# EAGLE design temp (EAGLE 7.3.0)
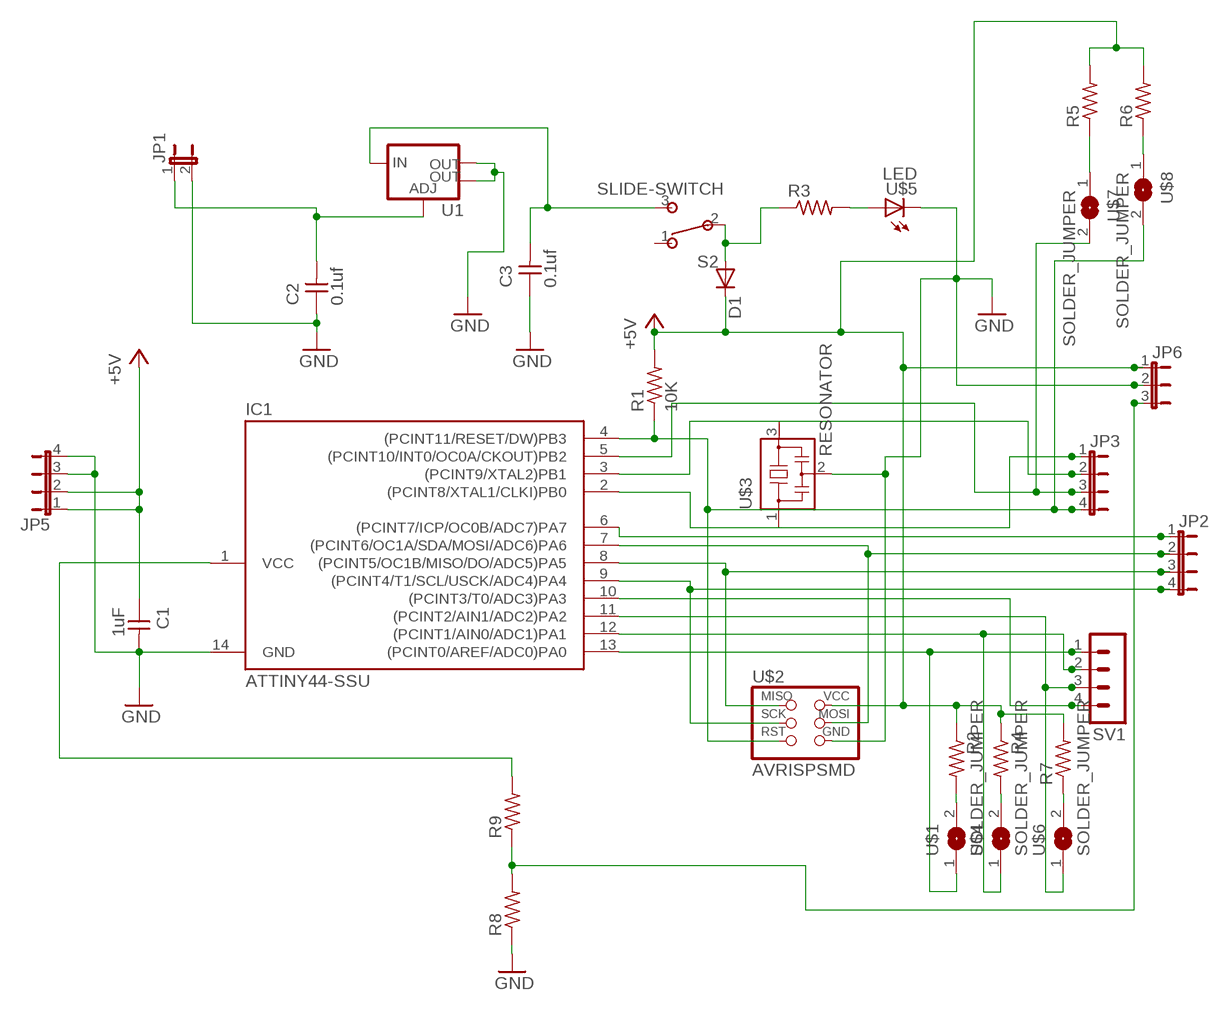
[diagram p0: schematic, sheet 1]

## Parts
C1  1uF  CAP-UNPOLARIZED  [C1206]
C2  0.1uf  CAP-UNPOLARIZED  [C1206]
C3  0.1uf  CAP-UNPOLARIZED  [C1206]
D1  DIODESOD123  [SOD123]
IC1  ATTINY44-SSU  [SOIC14]
JP1  JP1E  [JP1]
JP2  JP4E  [JP4]
JP3  JP4E  [JP4]
JP5  JP4E  [JP4]
JP6  JP2W  [JP2W]
R1  10K  RES-US1206  [R1206]
R2  RES-US1206FAB  [R1206FAB]
R3  RES-US1206  [R1206]
R4  RES-US1206FAB  [R1206FAB]
R5  RES-US1206FAB  [R1206FAB]
R6  RES-US1206FAB  [R1206FAB]
R7  RES-US1206FAB  [R1206FAB]
R8  RES-US1206FAB  [R1206FAB]
R9  RES-US1206FAB  [R1206FAB]
S2  SLIDE-SWITCH  [AYZ0102AGRLC]
SV1  MA04-1  [MA04-1]
U1  V_REG_LM1117SOT223  [SOT223]
U$1  SOLDER_JUMPER  [SJFAB]
U$2  AVRISPSMD  [2X03SMD]
U$3  RESONATOR  [EFOBM]
U$4  SOLDER_JUMPER  [SJFAB]
U$5  LED  [LED1206]
U$6  SOLDER_JUMPER  [SJFAB]
U$7  SOLDER_JUMPER  [SJFAB]
U$8  SOLDER_JUMPER  [SJFAB]

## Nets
+5V: C1.1 D1.CATHODE(C) IC1.1(VCC) JP5.1 JP5.2 JP6.1 R1.2 R2.1 R4.1 R5.2 R6.2 R7.2 R9.2 U$2.2(VCC)
GND: C1.2 C2.1 C3.1 IC1.14(GND) JP1.2 JP5.3 JP5.4 JP6.2 R8.1 U1.2(OUT) U1.4(OUT) U$2.6(GND) U$3.2 U$5.2(C)
N$1: IC1.2((PCINT8/XTAL1/CLKI)PB0) JP3.1 U$3.1
N$2: IC1.8((PCINT5/OC1B/MISO/DO/ADC5)PA5) JP2.3 U$2.1(MISO)
N$3: IC1.3((PCINT9/XTAL2)PB1) JP3.2 U$3.3
N$4: IC1.5((PCINT10/INT0/OC0A/CKOUT)PB2) JP3.3 U$7.2
N$5: IC1.4((PCINT11/RESET/DW)PB3) JP3.4 R1.1 U$2.5(RST) U$8.2
N$6: IC1.9((PCINT4/T1/SCL/USCK/ADC4)PA4) JP2.4 U$2.3(SCK)
N$7: IC1.7((PCINT6/OC1A/SDA/MOSI/ADC6)PA6) JP2.2 U$2.4(MOSI)
N$8: IC1.13((PCINT0/AREF/ADC0)PA0) SV1.1 U$1.1
N$9: IC1.12((PCINT1/AIN0/ADC1)PA1) SV1.2 U$4.1
N$10: IC1.11((PCINT2/AIN1/ADC2)PA2) SV1.3 U$6.1
N$11: IC1.10((PCINT3/T0/ADC3)PA3) SV1.4
N$12: C2.2 JP1.1 U1.1(ADJ)
N$13: C3.2 S2.3 U1.3(IN)
N$14: IC1.6((PCINT7/ICP/OC0B/ADC7)PA7) JP2.1
N$15: JP6.3 R8.2 R9.1
N$16: D1.ANODE(A) R3.1 S2.2
N$17: R3.2 U$5.1(A)
N$18: R2.2 U$1.2
N$19: R5.1 U$7.1
N$20: R6.1 U$8.1
N$21: R4.2 U$4.2
N$22: R7.1 U$6.2
Unconnected: S2.1

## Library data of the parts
C1-C3 = fab:CAP-UNPOLARIZED
D1 = fab:DIODE: DIODE
IC1 = fab:ATTINY44
JP1 = jumper:JP1E: JUMPER
JP2 JP3 JP5 = jumper:JP4E: JUMPER
JP6 = jumper:JP2W: JUMPER
R1-R9 = fab:RES-US: Resistor (US Symbol)
S2 = fab:SLIDE-SWITCH: SMD slide-switch AYZ0102AGRLC as found in the fablab inventory. Includes the mounting holes. Made by Zaerc.
SV1 = con-lstb:MA04-1: PIN HEADER; OC_FARNELL: unknown; OC_NEWARK: unknown
U1 = fab:V_REG_LM1117: Voltage Regulator LM1117 Standard adjustable voltage regulator but in SMD form. Spark Fun Electronics SKU : COM-00595; PROD_ID: VREG-08170
U$1 U$4 U$6-U$8 = fab:SOLDER_JUMPER
U$2 = fab:AVRISP
U$3 = fab:RESONATOR
U$5 = fab:LED: LED

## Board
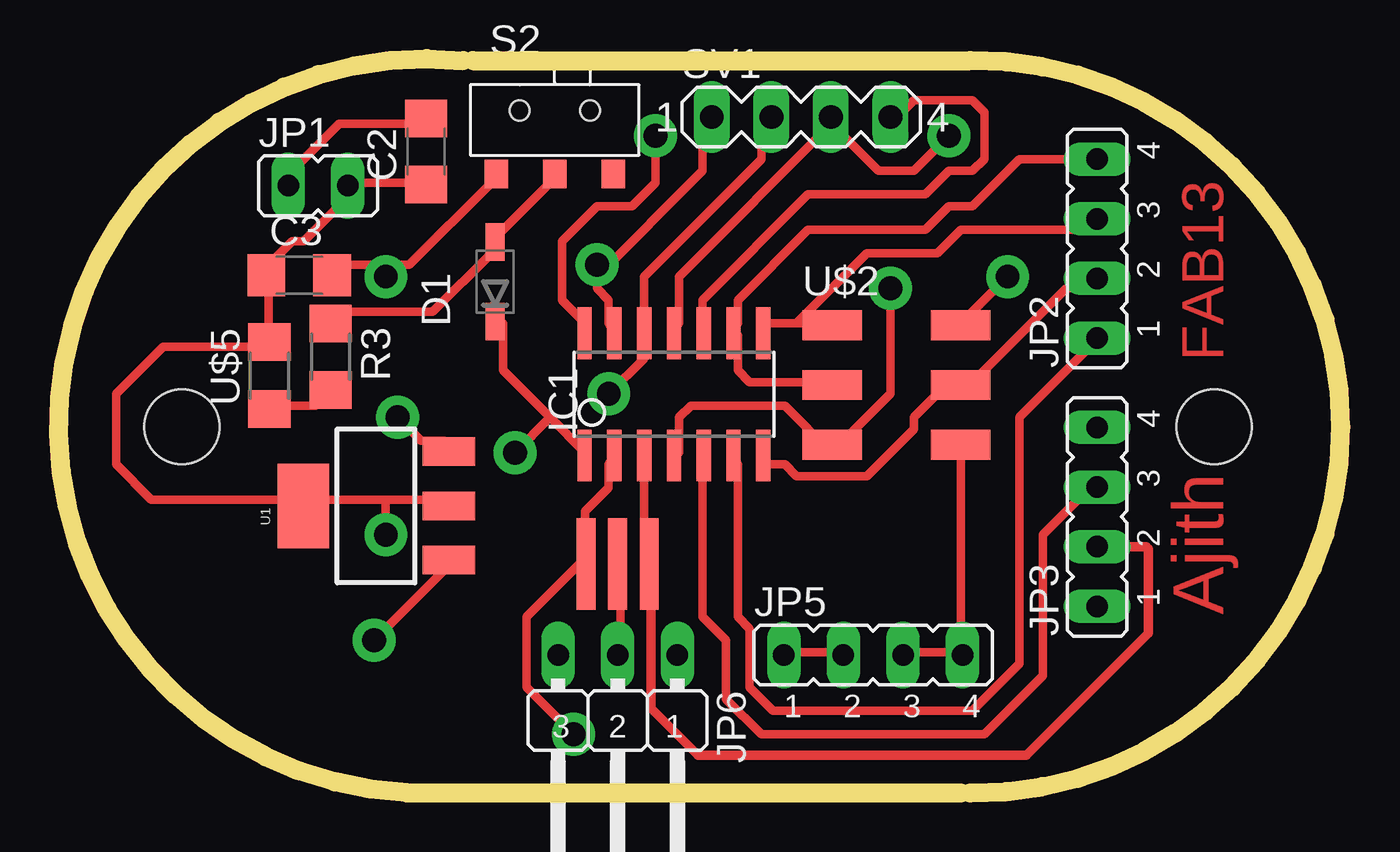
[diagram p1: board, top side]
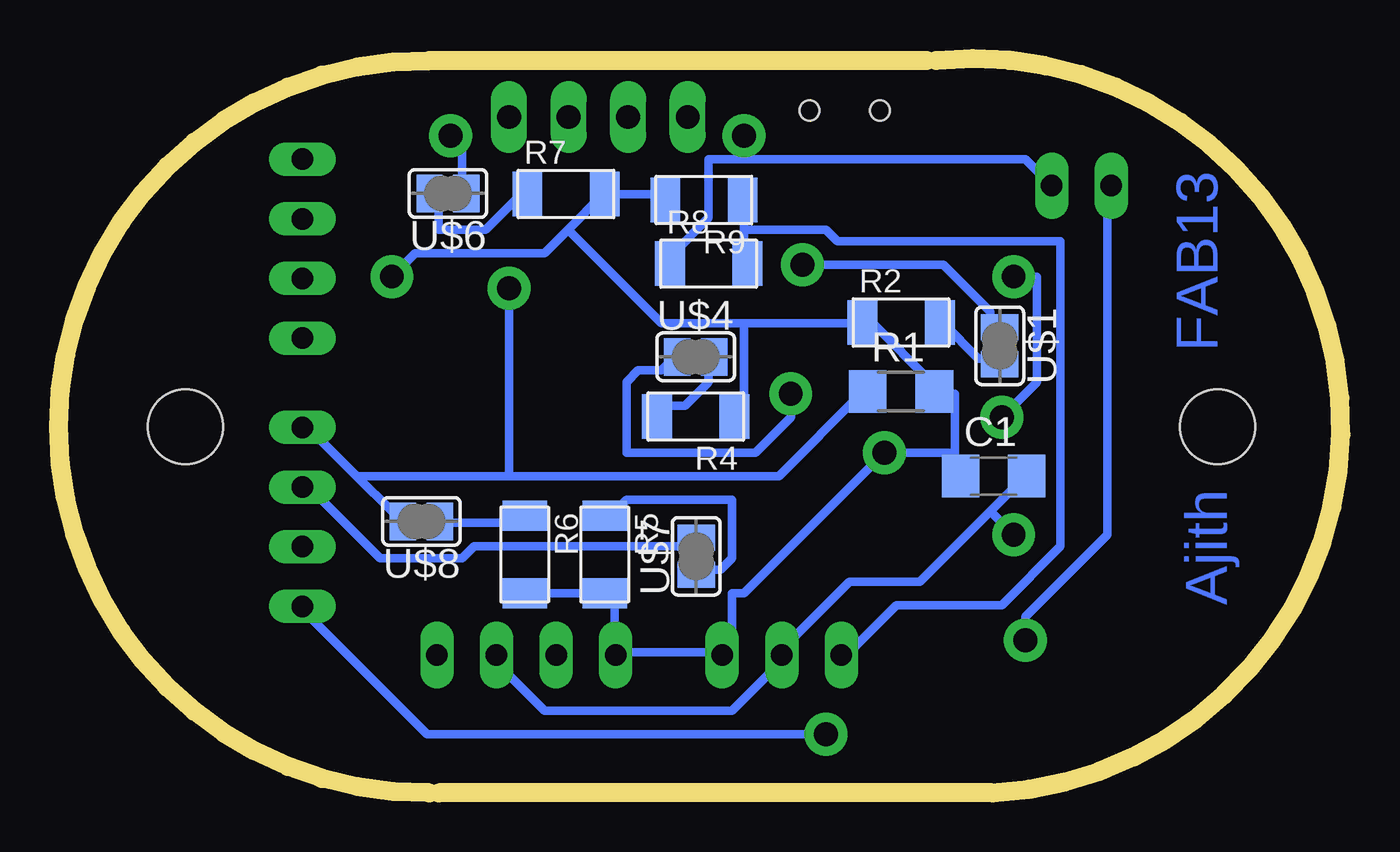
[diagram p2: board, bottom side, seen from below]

Size 54.65 x 31.28 mm. Coordinates in mm from the lower left corner, seen from the top.
Outline: 17.64,31.2 38.84,31.2 arc-181 38.84,0
Outline: 38.44,0 14.84,0 arc-183 17.24,31.2
Copper layers (1*16): Top 0.035mm / dielectric 1.5mm / Bottom 0.035mm
Design rules "default *": minimum track width 14mil, minimum drill 40mil, track to track 16mil, track to pad 16mil, pad to pad 16mil, via to via 16mil, smd to smd 16mil, copper to edge 40mil, drill to drill 16mil, minimum pad ring 10mil, minimum via ring 16mil, stop-mask expansion 4mil, vias tented up to drill 0mil, thermal gap 10mil
Holes 3.2 mm at 49.24,15.6 5.24,15.6

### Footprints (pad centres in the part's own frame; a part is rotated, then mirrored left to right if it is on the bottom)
C1206 = smd 1.6 x 1.8: 1 -1.4,0; 2 1.4,0
SOD123 = smd 1.6 x 0.8: ANODE 1.7,0; CATHODE -1.7,0
SOIC14 = smd 0.61 x 2.21: 1 -3.81,-2.603; 2 -2.54,-2.603; 3 -1.27,-2.603; 4 0,-2.603; 5 1.27,-2.603; 6 2.54,-2.603; 7 3.81,-2.603; 8 3.81,2.603; 9 2.54,2.603; 10 1.27,2.603; 11 0,2.603; 12 -1.27,2.603; 13 -2.54,2.603; 14 -3.81,2.603
JP1 = drill 0.914 long: 1 0,-1.27; 2 0,1.27
JP4 = drill 0.914 long: 1 -3.81,0; 2 -1.27,0; 3 1.27,0; 4 3.81,0
JP2W = drill 0.914 long: 1 -2.54,-1.27; 2 0,-1.27; 3 2.54,-1.27
R1206 = smd 1.6 x 1.803: 1 -1.422,0; 2 1.422,0
R1206FAB = smd 1.27 x 1.905: 1 -1.651,0; 2 1.651,0
AYZ0102AGRLC = smd 1 x 1.2: 1 2.5,-2.3; 2 0,-2.3; 3 -2.5,-2.3 | hole 0.85: -1.5,0.4; 1.5,0.4
MA04-1 = drill 1.016 long: 1 -3.81,0; 2 -1.27,0; 3 1.27,0; 4 3.81,0
SOT223 = smd 1.219 x 2.235: 1 -2.311,-3.099; 2 0,-3.099; 3 2.311,-3.099 | smd 3.6 x 2.2: 4 0,3.099
SJFAB = smd 1.118 x 1.6: 1 -0.787,0; 2 0.787,0
2X03SMD = smd 2.54 x 1.27: 1 -2.54,2.54; 2 2.92,2.54; 3 -2.54,0; 4 2.92,0; 5 -2.54,-2.54; 6 2.92,-2.54
EFOBM = smd 0.8 x 3.9: 1 -1.35,0; 2 0,0; 3 1.35,0
LED1206 = smd 1.6 x 1.803: 1 -1.422,0; 2 1.422,0

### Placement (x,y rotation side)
C1  14.79,13.5 0 bottom
C2  15.66,27.33 90 top
C3  10.25,22.06 0 top
D1  18.6,21.78 90 top
IC1  26.22,16.98 0 top
JP1  11.05,25.87 270 top
JP2  44.26,23.19 90 top
JP3  44.26,11.76 90 top
JP5  34.71,5.88 0 top
JP6  23.82,4.61 180 top
R1  18.74,17.1 0 bottom
R2  18.74,20.04 0 bottom
R3  11.59,18.58 270 top
R4  27.49,16.04 180 bottom
R5  31.37,10.16 270 bottom
R6  34.78,10.16 270 bottom
R7  33.02,25.52 0 bottom
R8  26.94,22.55 0 bottom
R9  27.14,25.26 180 bottom
S2  21.14,28.67 0 top
SV1  31.64,28.8 0 top
U1  13.52,12.23 90 top
U$1  14.53,19.05 270 bottom
U$2  35.51,17.38 0 top
U$3  23.82,9.76 0 top
U$4  27.49,18.58 0 bottom
U$5  8.98,17.78 90 top
U$6  38.05,25.54 180 bottom
U$7  27.47,10.08 90 bottom
U$8  39.18,11.57 180 bottom

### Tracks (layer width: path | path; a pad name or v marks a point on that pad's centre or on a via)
+5V  (via drill 1.02)
  Top 0.356: v40.44,22 38.44,20 U$2.2 | JP5.2 33.44,6 30.94,6 JP5.1 | 20.94,16 22.44,14.5 IC1.1 | 20.94,16 18.94,18 18.94,20 D1.CATHODE | v19.44,14.5 20.94,16
  Bottom 0.356: R9.2 28.94,25.5 30.94,25.5 R7.2 31.44,25.5 32.94,24 | v40.44,22 39.44,23 33.94,23 32.94,24 | R6.2 34.44,8.5 31.44,8.5 R5.2 30.94,8.5 30.94,6 JP5.1 30.44,6 26.44,6 JP6.1 25.94,6 25.94,8.5 25.44,8.5 v19.44,14.5 16.44,14.5 | 16.44,14.5 16.44,17 16.94,17 R1.2 17.44,17.5 19.94,20 R2.1 20.44,20 25.44,20 | 16.44,14.5 16.44,13.5 C1.1 | 25.44,20 25.44,16.5 R4.1 | 32.94,24 28.94,20 25.44,20
GND  (via drill 1.02)
  Top 0.356: 38.44,6 38.44,14.5 U$2.6 | 38.44,6 36.44,6 JP5.3 | 38.44,6 JP5.4 | U$3.2 23.94,9.5 23.94,6 JP6.2 | 13.94,12.5 10.44,12.5 U1.4 9.94,12.5 3.94,12.5 2.44,14 2.44,17 4.44,19 8.94,19 U$5.2 8.94,19.5 8.94,22 C3.1 8.94,22.5 9.94,23.5 10.44,23.5 12.44,25.5 JP1.2 12.44,26 15.44,26 C2.1 | 13.94,12.5 16.44,12.5 U1.2 | v25.44,28 25.44,26 24.44,25 22.94,25 21.44,23.5 21.44,21 22.44,20 IC1.14 | 13.94,12.5 v13.94,11
  Bottom 0.356: 14.94,12 17.94,9 20.94,9 23.94,6 JP6.2 23.94,5.5 25.94,3.5 33.94,3.5 35.94,5.5 JP5.3 | 14.94,12 13.44,13.5 C1.2 | 25.44,27 13.44,27 12.44,26 JP1.2 | 25.44,27 26.94,27 26.94,24.5 28.44,23 R8.1 | 25.44,27 v25.44,28 | v13.94,11 14.94,12
N$1  (via drill 1.02)
  Top 0.356: 22.44,10 22.44,12 23.44,13 23.44,14 IC1.2 | v21.94,2.5 19.94,4.5 19.94,7.5 22.44,10 | 22.44,10 U$3.1
  Bottom 0.356: v21.94,2.5 38.94,2.5 43.94,7.5 JP3.1
N$2
  Top 0.356: 31.44,20 32.94,20 U$2.1 | 31.44,20 29.94,20 IC1.8 | 31.44,20 34.44,23 37.44,23 38.44,24 43.94,24 JP2.3
N$3
  Top 0.356: IC1.3 24.94,14 24.94,10 U$3.3
  Top 0.406: U$3.3 25.24,9.69 25.24,3.6 27.24,1.6 41.24,1.6 46.44,6.8 46.44,10.4 46.35,10.49 JP3.2
N$4
  Top 0.356: IC1.5 27.44,14 27.44,7.5 28.44,6.5 28.44,4 29.94,2.5 39.44,2.5 41.94,5 41.94,11 43.94,13 JP3.3
  Bottom 0.356: U$7.2 27.94,10.5 36.94,10.5 37.44,10 40.94,10 43.94,13 JP3.3
N$5  (via drill 1.02)
  Top 0.356: IC1.4 26.44,14.5 26.44,16 26.94,16.5 30.94,16.5 32.94,14.5 U$2.5 33.44,15 35.44,17 v35.44,21.5
  Bottom 0.356: 41.94,13.5 43.94,15.5 JP3.4 | 41.94,13.5 40.44,12 U$8.2 | 41.94,13.5 35.44,13.5 | 35.44,13.5 23.94,13.5 20.44,17 R1.1 | 35.44,13.5 v35.44,21.5
N$6
  Top 0.356: U$2.3 32.94,17.5 29.44,17.5 28.94,18 28.94,19.5 IC1.9 28.94,20 28.94,21 31.94,24 36.94,24 37.94,25 38.94,25 40.94,27 JP2.4
N$7
  Top 0.356: IC1.7 29.94,14 30.94,14 31.44,13.5 34.44,13.5 36.44,15.5 36.44,16 37.94,17.5 U$2.4 38.44,17 42.94,21.5 43.94,21.5 JP2.2
N$8  (via drill 1.02)
  Top 0.356: 22.94,22 22.94,21.5 23.44,21 23.44,20 IC1.13 | 22.94,22 27.44,26.5 27.44,28.5 SV1.1 | 22.94,22 v22.94,22.5
  Bottom 0.356: v22.94,22.5 16.94,22.5 14.94,20.5 14.94,20 U$1.1
N$9  (via drill 1.02)
  Top 0.356: v23.44,17 24.94,18.5 24.94,19.5 IC1.12 24.94,20 24.94,22 29.94,27 29.94,28.5 SV1.2
  Bottom 0.356: v23.44,17 23.44,16 24.94,14.5 30.44,14.5 30.44,17.5 29.94,18 28.94,18 28.44,18.5 U$4.1
N$10  (via drill 1.02)
  Top 0.356: v37.94,28 36.44,26.5 34.94,26.5 32.94,28.5 | 32.94,28.5 26.44,22 26.44,20 IC1.11 | 32.94,28.5 SV1.3
  Bottom 0.356: v37.94,28 37.44,28 37.44,26 U$6.1
N$11
  Top 0.356: IC1.10 27.44,20 27.44,21 31.94,25.5 36.94,25.5 37.94,26.5 38.94,26.5 39.44,27 39.44,29 38.94,29.5 36.44,29.5 35.94,29 SV1.4
N$12  (via drill 1.02)
  Top 0.356: C2.2 15.44,28.5 11.94,28.5 9.44,26 JP1.1 | v13.44,6.5 16.44,9.5 U1.1
  Bottom 0.356: v13.44,6.5 13.44,7.5 9.94,11 9.94,25.5 JP1.1
N$13  (via drill 1.02)
  Top 0.356: 13.94,22.5 11.94,22.5 C3.2 | 13.94,22.5 14.94,22.5 18.44,26 S2.3 | v14.44,16 15.44,15 16.44,15 U1.3 | 13.94,22.5 v13.94,22
  Bottom 0.356: v14.44,16 12.94,17.5 12.94,22 v13.94,22
N$14
  Top 0.356: IC1.6 28.94,14 28.94,7.5 29.44,7 29.44,4.5 30.44,3.5 38.94,3.5 40.94,5.5 40.94,16 43.94,19 JP2.1
N$15
  Bottom 0.356: 25.44,24 25.44,25 R9.1 | 25.44,24 25.44,23 R8.2 | 25.44,24 21.94,24 21.44,23.5 11.94,23.5 11.94,10.5 14.44,8 18.94,8 20.94,6 JP6.3
N$16
  Top 0.356: S2.2 20.94,26 18.44,23.5 D1.ANODE 18.44,23 15.94,20.5 11.94,20.5 R3.1
N$17
  Top 0.356: U$5.1 9.44,16.5 10.94,16.5 11.44,17 R3.2
N$18
  Bottom 0.356: U$1.2 14.94,18.5 15.44,18.5 16.94,20 R2.2
N$19
  Bottom 0.356: U$7.1 27.44,9.5 26.44,9.5 25.94,10 25.94,12.5 30.44,12.5 30.94,12 R5.1
N$20
  Bottom 0.356: U$8.1 37.94,11.5 34.94,11.5 R6.1
N$21
  Bottom 0.356: U$4.2 26.94,18.5 26.94,17.5 27.94,16.5 28.94,16.5 R4.2
N$22
  Bottom 0.356: U$6.2 38.44,25.5 38.44,24 36.44,24 34.94,25.5 R7.1

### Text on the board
Top: FAB13 | Ajith
Bottom: FAB13 | Ajith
